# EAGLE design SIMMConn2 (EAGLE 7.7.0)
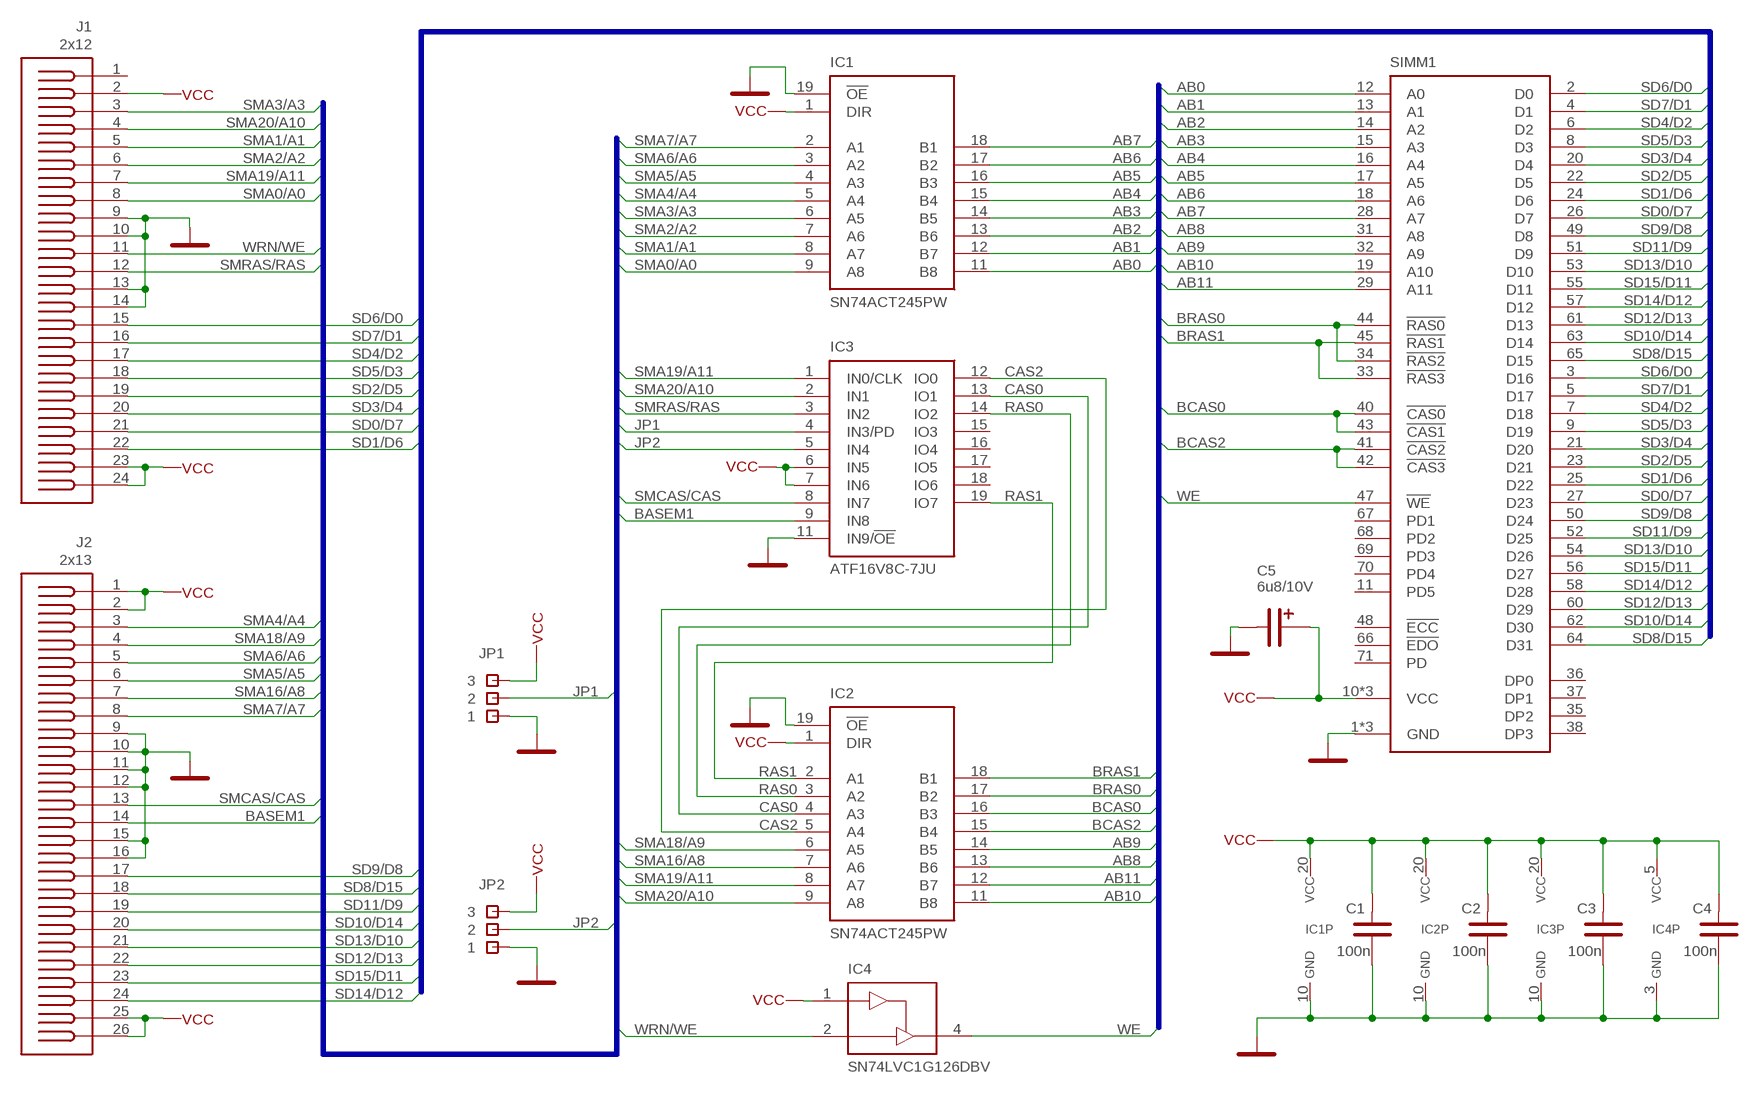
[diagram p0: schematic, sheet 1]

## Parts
C1  100n  CK-SMD-0805  [CK-0805]
C2  100n  CK-SMD-0805  [CK-0805]
C3  100n  CK-SMD-0805  [CK-0805]
C4  100n  CK-SMD-0805  [CK-0805]
C5  6u8/10V  CT-SMD-B  [CT-SMD-B]
IC1  SN74ACT245PW  74245-PW  [TSSOP20]
IC2  SN74ACT245PW  74245-PW  [TSSOP20]
IC3  ATF16V8C-7JU  ATF16V8C  [PLCC20SKT]
IC4  SN74LVC1G126DBV  74-1G126DBV  [SOT23-5]
J1  2x12  20-Z2R24T  [20-Z2R24T]
J2  2x13  20-Z2R26T  [20-Z2R26T]
JP1  JMP1-3  [JMP3-1]
JP2  JMP1-3  [JMP3-1]
SIMM1  SIMM72  [SIMM72A]

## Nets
AB0: IC1.11(B8) SIMM1.12(A0)
AB1: IC1.12(B7) SIMM1.13(A1)
AB2: IC1.13(B6) SIMM1.14(A2)
AB3: IC1.14(B5) SIMM1.15(A3)
AB4: IC1.15(B4) SIMM1.16(A4)
AB5: IC1.16(B3) SIMM1.17(A5)
AB6: IC1.17(B2) SIMM1.18(A6)
AB7: IC1.18(B1) SIMM1.28(A7)
AB8: IC2.13(B6) SIMM1.31(A8)
AB9: IC2.14(B5) SIMM1.32(A9)
AB10: IC2.11(B8) SIMM1.19(A10)
AB11: IC2.12(B7) SIMM1.29(A11)
BASEM1: IC3.9(IN8) J2.14
BCAS0: IC2.16(B3) SIMM1.40(!CAS0) SIMM1.43(!CAS1)
BCAS2: IC2.15(B4) SIMM1.41(!CAS2) SIMM1.42(!CAS3)
BRAS0: IC2.17(B2) SIMM1.34(!RAS2) SIMM1.44(!RAS0)
BRAS1: IC2.18(B1) SIMM1.33(!RAS3) SIMM1.45(!RAS1)
CAS0: IC2.4(A3) IC3.13(IO1)
CAS2: IC2.5(A4) IC3.12(IO0)
GND: C1.1 C2.1 C3.1 C4.1 C5.K IC1.10(GND) IC1.19(!OE) IC2.10(GND) IC2.19(!OE) IC3.10(GND) IC3.11(IN9/!OE) IC4.3(GND) J1.9 J1.10 J1.13 J1.14 J2.9 J2.10 J2.11 J2.12 J2.15 J2.16 JP1.1 JP2.1 SIMM1.1(GND) SIMM1.39(GND) SIMM1.72(GND)
JP1: IC3.4(IN3/PD) JP1.2
JP2: IC3.5(IN4) JP2.2
RAS0: IC2.3(A2) IC3.14(IO2)
RAS1: IC2.2(A1) IC3.19(IO7)
SD0/D7: J1.21 SIMM1.26(D7) SIMM1.27(D23)
SD1/D6: J1.22 SIMM1.24(D6) SIMM1.25(D22)
SD2/D5: J1.19 SIMM1.22(D5) SIMM1.23(D21)
SD3/D4: J1.20 SIMM1.20(D4) SIMM1.21(D20)
SD4/D2: J1.17 SIMM1.6(D2) SIMM1.7(D18)
SD5/D3: J1.18 SIMM1.8(D3) SIMM1.9(D19)
SD6/D0: J1.15 SIMM1.2(D0) SIMM1.3(D16)
SD7/D1: J1.16 SIMM1.4(D1) SIMM1.5(D17)
SD8/D15: J2.18 SIMM1.64(D31) SIMM1.65(D15)
SD9/D8: J2.17 SIMM1.49(D8) SIMM1.50(D24)
SD10/D14: J2.20 SIMM1.62(D30) SIMM1.63(D14)
SD11/D9: J2.19 SIMM1.51(D9) SIMM1.52(D25)
SD12/D13: J2.22 SIMM1.60(D29) SIMM1.61(D13)
SD13/D10: J2.21 SIMM1.53(D10) SIMM1.54(D26)
SD14/D12: J2.24 SIMM1.57(D12) SIMM1.58(D28)
SD15/D11: J2.23 SIMM1.55(D11) SIMM1.56(D27)
SMA0/A0: IC1.9(A8) J1.8
SMA1/A1: IC1.8(A7) J1.5
SMA2/A2: IC1.7(A6) J1.6
SMA3/A3: IC1.6(A5) J1.3
SMA4/A4: IC1.5(A4) J2.3
SMA5/A5: IC1.4(A3) J2.6
SMA6/A6: IC1.3(A2) J2.5
SMA7/A7: IC1.2(A1) J2.8
SMA16/A8: IC2.7(A6) J2.7
SMA18/A9: IC2.6(A5) J2.4
SMA19/A11: IC2.8(A7) IC3.1(IN0/CLK) J1.7
SMA20/A10: IC2.9(A8) IC3.2(IN1) J1.4
SMCAS/CAS: IC3.8(IN7) J2.13
SMRAS/RAS: IC3.3(IN2) J1.12
VCC: C1.2 C2.2 C3.2 C4.2 C5.A IC1.1(DIR) IC1.20(VCC) IC2.1(DIR) IC2.20(VCC) IC3.6(IN5) IC3.7(IN6) IC3.20(VCC) IC4.1(OE) IC4.5(VCC) J1.2 J1.23 J1.24 J2.1 J2.2 J2.25 J2.26 JP1.3 JP2.3 SIMM1.10(VCC) SIMM1.30(VCC) SIMM1.59(VCC)
WE: IC4.4(Y) SIMM1.47(!WE)
WRN/WE: IC4.2(A) J1.11
Unconnected: IC3.15(IO3) IC3.16(IO4) IC3.17(IO5) IC3.18(IO6) J1.1 SIMM1.11(PD5) SIMM1.35(DP2) SIMM1.36(DP0) SIMM1.37(DP1) SIMM1.38(DP3) SIMM1.48(!ECC) SIMM1.66(!EDO) SIMM1.67(PD1) SIMM1.68(PD2) SIMM1.69(PD3) SIMM1.70(PD4) SIMM1.71(PD)

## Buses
D:SD6/D0,SD7/D1,SD4/D2,SD5/D3,SD2/D5,SD3/D4,SD0/D7,SD1/D6,SD9/D8,SD8/D15,SD11/D9,SD10/D14,SD13/D10,SD12/D13,SD15/D11,SD14/D12
A:SMA3/A3,SMA20/A10,SMA1/A1,SMA2/A2,SMA19/A11,SMA0/A0,WRN/WE,SMRAS/RAS,SMA4/A4,SMA18/A9,SMA6/A6,SMA5/A5,SMA16/A8,SMA7/A7,SMCAS/CAS,BASEM1,PD1,PD2,JP1,JP2
B:AB[0..11],BCAS0,BCAS2,BRAS0,BRAS1,WE

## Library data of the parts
C1-C4 = PASIV:CK-SMD: SMD keramické vícevrstvé kondenzátory
C5 = PASIV:CT-SMD: SMD tantalové kondenzátory
IC1 IC2 = IC:74245
IC3 = MEMORY:ATF16V8C
IC4 = IC:74-1G126
J1 = CONNEC:20-Z2R24T
J2 = CONNEC:20-Z2R26T
JP1 JP2 = KONSTR:JMP1-3
SIMM1 = CONNEC:SIMM72

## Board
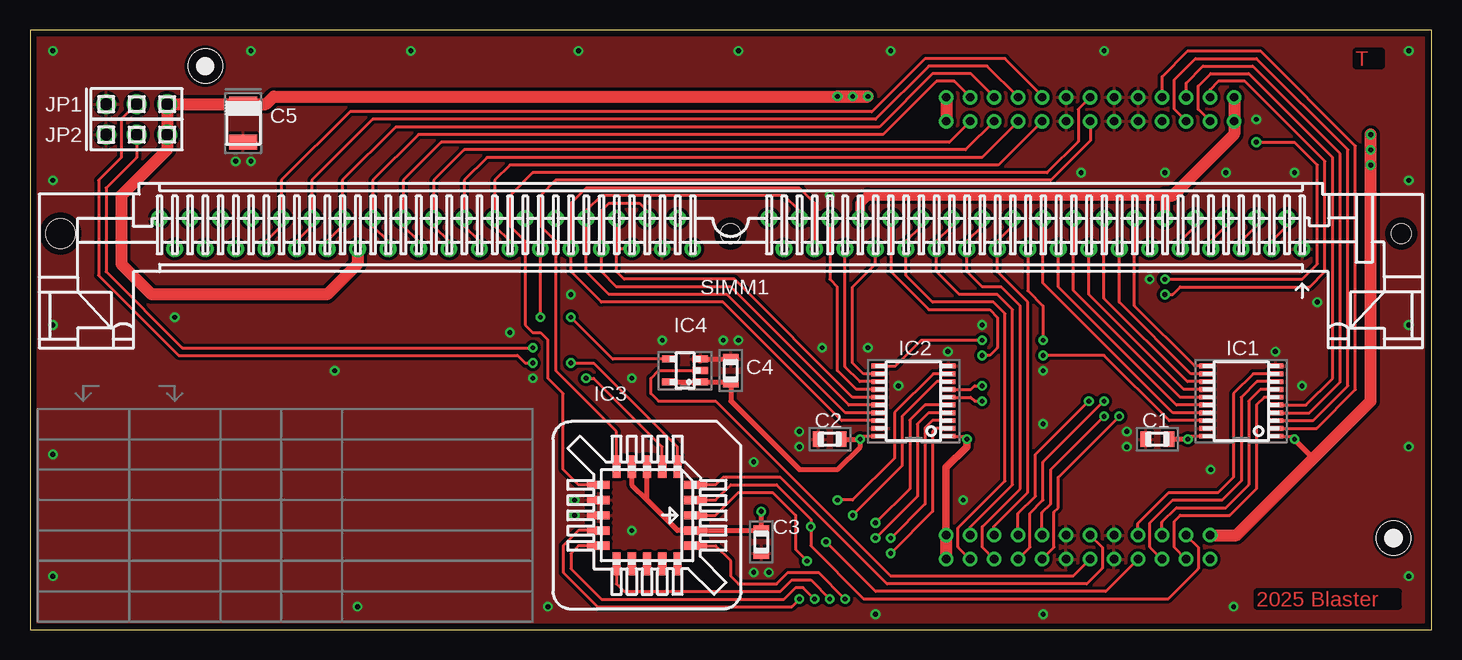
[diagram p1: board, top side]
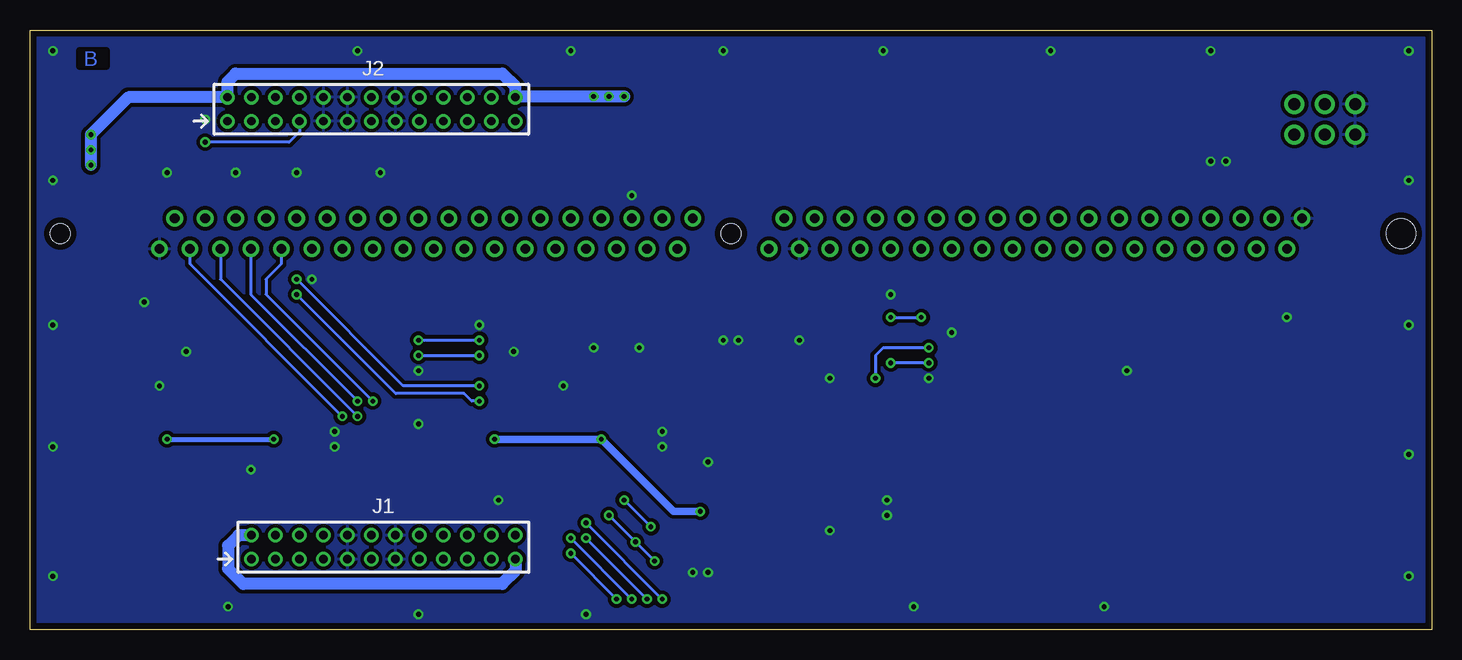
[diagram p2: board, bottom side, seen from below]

Size 116.84 x 50 mm. Coordinates in mm from the lower left corner, seen from the top.
Outline: 0,0 116.84,0 116.84,50 0,50 0,0
Copper layers (1*16): Top 0.035mm / dielectric 1.5mm / Bottom 0.035mm
Design rules "default *": minimum track width 10mil, minimum drill 15mil, track to track 8mil, track to pad 8mil, pad to pad 8mil, via to via 8mil, smd to smd 8mil, copper to edge 20mil, drill to drill 8mil, minimum pad ring 10mil, minimum via ring 8mil, stop-mask expansion 0mil, vias tented up to drill 20mil, thermal gap 10mil
tRestrict: area 110.5,47 to 112.7,48.3
bRestrict: area 110.5,47 to 112.7,48.3

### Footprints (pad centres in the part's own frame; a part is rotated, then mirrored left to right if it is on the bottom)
CK-0805 = smd 0.889 x 1.295: 1 -0.953,0; 2 0.953,0
CT-SMD-B = smd 1.245 x 2.311: A -1.587,0; K 1.587,0
TSSOP20 = smd 0.4 x 1.2: 1 -2.925,-2.9; 2 -2.275,-2.9; 3 -1.625,-2.9; 4 -0.975,-2.9; 5 -0.325,-2.9; 6 0.325,-2.9; 7 0.975,-2.9; 8 1.625,-2.9; 9 2.275,-2.9; 10 2.925,-2.9; 11 2.925,2.9; 12 2.275,2.9; 13 1.625,2.9; 14 0.975,2.9; 15 0.325,2.9; 16 -0.325,2.9; 17 -0.975,2.9; 18 -1.625,2.9; 19 -2.275,2.9; 20 -2.925,2.9
PLCC20SKT = smd 0.7 x 1.91: 1 0,4.06; 2 -1.27,4.06; 3 -2.54,4.06; 9 -2.54,-4.06; 10 -1.27,-4.06; 11 0,-4.06; 12 1.27,-4.06; 13 2.54,-4.06; 19 2.54,4.06; 20 1.27,4.06 | smd 1.91 x 0.7: 4 -4.06,2.54; 5 -4.06,1.27; 6 -4.06,0; 7 -4.06,-1.27; 8 -4.06,-2.54; 14 4.06,-2.54; 15 4.06,-1.27; 16 4.06,0; 17 4.06,1.27; 18 4.06,2.54
SOT23-5 = smd 0.584 x 1.27: 1 0.953,1.27; 2 0,1.27; 3 -0.953,1.27; 4 -0.953,-1.27; 5 0.953,-1.27
20-Z2R24T = drill 0.7 pad 1.2: 1 0,0; 2 0,-2; 3 -2,0; 4 -2,-2; 5 -4,0; 6 -4,-2; 7 -6,0; 8 -6,-2; 9 -8,0; 10 -8,-2; 11 -10,0; 12 -10,-2; 13 -12,0; 14 -12,-2; 15 -14,0; 16 -14,-2; 17 -16,0; 18 -16,-2; 19 -18,0; 20 -18,-2; 21 -20,0; 22 -20,-2; 23 -22,0; 24 -22,-2
20-Z2R26T = drill 0.7 pad 1.2: 1 0,0; 2 0,-2; 3 -2,0; 4 -2,-2; 5 -4,0; 6 -4,-2; 7 -6,0; 8 -6,-2; 9 -8,0; 10 -8,-2; 11 -10,0; 12 -10,-2; 13 -12,0; 14 -12,-2; 15 -14,0; 16 -14,-2; 17 -16,0; 18 -16,-2; 19 -18,0; 20 -18,-2; 21 -20,0; 22 -20,-2; 23 -22,0; 24 -22,-2; 25 -24,0; 26 -24,-2
JMP3-1 = drill 1 pad 1.676: 1 0,0; 2 2.54,0; 3 5.08,0
SIMM72A = drill 0.8 pad 1.4: 1 0,0; 2 -1.27,2.54; 3 -2.54,0; 4 -3.81,2.54; 5 -5.08,0; 6 -6.35,2.54; 7 -7.62,0; 8 -8.89,2.54; 9 -10.16,0; 10 -11.43,2.54; 11 -12.7,0; 12 -13.97,2.54; 13 -15.24,0; 14 -16.51,2.54; 15 -17.78,0; 16 -19.05,2.54; 17 -20.32,0; 18 -21.59,2.54; 19 -22.86,0; 20 -24.13,2.54; 21 -25.4,0; 22 -26.67,2.54; 23 -27.94,0; 24 -29.21,2.54; 25 -30.48,0; 26 -31.75,2.54; 27 -33.02,0; 28 -34.29,2.54; 29 -35.56,0; 30 -36.83,2.54; 31 -38.1,0; 32 -39.37,2.54; 33 -40.64,0; 34 -41.91,2.54; 35 -43.18,0; 36 -44.45,2.54; 37 -50.8,0; 38 -52.07,2.54; 39 -53.34,0; 40 -54.61,2.54; 41 -55.88,0; 42 -57.15,2.54; 43 -58.42,0; 44 -59.69,2.54; 45 -60.96,0; 46 -62.23,2.54; 47 -63.5,0; 48 -64.77,2.54; 49 -66.04,0; 50 -67.31,2.54; 51 -68.58,0; 52 -69.85,2.54; 53 -71.12,0; 54 -72.39,2.54; 55 -73.66,0; 56 -74.93,2.54; 57 -76.2,0; 58 -77.47,2.54; 59 -78.74,0; 60 -80.01,2.54; 61 -81.28,0; 62 -82.55,2.54; 63 -83.82,0; 64 -85.09,2.54; 65 -86.36,0; 66 -87.63,2.54; 67 -88.9,0; 68 -90.17,2.54; 69 -91.44,0; 70 -92.71,2.54; 71 -93.98,0; 72 -95.25,2.54 | hole 2.45: -103.51,1.27 | hole 1.65: -47.63,1.27; 8.26,1.27

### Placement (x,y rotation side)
C1  93.98,15.88 0 top
C2  66.67,15.88 0 top
C3  60.96,7.3 90 top
C4  58.42,21.59 270 top
C5  17.78,42.23 270 top
IC1  100.97,19.05 90 top
IC2  73.66,19.05 90 top
IC3  51.44,9.53 270 top
IC4  54.61,21.59 270 top
J1  98.37,5.87 180 bottom
J2  100.38,42.39 180 bottom
JP1  6.35,43.81 0 top
JP2  6.35,41.27 0 top
REF1  [REF-K]  14.61,46.99 0 top
REF2  [REF-K]  113.67,7.62 0 top
SIMM1  106.05,31.75 0 top

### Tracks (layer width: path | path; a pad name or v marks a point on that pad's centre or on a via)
AB0
  Top 0.254: SIMM1.12 92.08,26.99 97.09,21.98 IC1.11
AB1
  Top 0.254: SIMM1.13 90.81,27.3 96.78,21.32 IC1.12
AB2
  Top 0.254: SIMM1.14 89.53,27.62 96.48,20.68 IC1.13
AB3
  Top 0.254: SIMM1.15 88.27,27.94 96.18,20.02 IC1.14
AB4
  Top 0.254: SIMM1.16 87,28.26 95.88,19.38 IC1.15
AB5
  Top 0.254: SIMM1.17 85.72,28.57 95.58,18.73 IC1.16
AB6
  Top 0.254: SIMM1.18 84.45,28.89 95.27,18.07 IC1.17
AB7  (via drill 0.4)
  Top 0.254: v84.45,22.86 89.53,22.86 94.97,17.43 IC1.18 | SIMM1.28 71.75,29.84 74.93,26.67 80.01,26.67 80.64,26.04 80.64,23.5 80.01,22.86 v79.38,22.86
  Bottom 0.254: v84.45,22.86 v79.38,22.86
AB8
  Top 0.254: SIMM1.31 67.94,21.91 69.18,20.68 IC2.13
AB9
  Top 0.254: SIMM1.32 66.67,29.21 67.31,28.57 67.31,21.59 68.88,20.02 IC2.14
AB10  (via drill 0.4)
  Top 0.254: SIMM1.19 83.19,28.26 84.45,26.99 v84.45,24.13 | IC2.11 72.14,21.98 74.3,24.13 v79.38,24.13
  Bottom 0.254: v84.45,24.13 v79.38,24.13
AB11
  Top 0.254: SIMM1.29 70.48,30.48 68.58,28.57 68.58,22.23 69.48,21.32 IC2.12
BASEM1
  Top 0.254: IC3.9 45.72,12.06 44.45,13.34 44.45,19.68 43.18,20.95 43.18,24.13 42.55,24.77 41.91,24.77 41.27,25.4 41.27,32.38 40.01,33.66 40.01,36.2 41.91,38.1 84.77,38.1 87.38,40.7 87.38,43.39 J2.14
BCAS0
  Top 0.254: SIMM1.40 51.44,34.92 50.8,35.56 48.26,35.56 47.62,34.92 SIMM1.43 47.62,29.84 48.9,28.57 58.42,28.57 68.27,18.73 IC2.16
BCAS2
  Top 0.254: 48.9,31.75 48.9,29.84 49.53,29.21 58.74,29.21 68.57,19.38 IC2.15 | 48.9,31.75 SIMM1.42 | SIMM1.41 48.9,31.75
BRAS0
  Top 0.254: SIMM1.34 64.14,34.92 62.87,36.2 47.62,36.2 46.35,34.92 SIMM1.44 46.35,29.84 48.26,27.94 58.1,27.94 67.97,18.07 IC2.17
BRAS1
  Top 0.254: SIMM1.33 65.41,35.56 64.14,36.83 46.35,36.83 45.09,35.56 SIMM1.45 45.09,29.84 47.62,27.3 57.78,27.3 67.67,17.43 IC2.18
CAS0  (via drill 0.4)
  Top 0.254: IC3.13 45.72,6.99 45.09,6.35 45.09,5.08 47.62,2.54 62.87,2.54 63.82,3.49 64.45,3.49 v65.41,2.54 | IC2.4 74.91,18.07 73.98,17.14 73.98,11.11 v70.48,7.62
  Bottom 0.254: v70.48,7.62 v65.41,2.54
CAS2  (via drill 0.4)
  Top 0.254: IC3.12 45.72,8.26 44.45,6.99 44.45,4.76 47.31,1.91 63.5,1.91 v64.14,2.54 | IC2.5 74.61,18.73 73.34,17.46 73.34,11.75 v70.48,8.89
  Bottom 0.254: v70.48,8.89 v64.14,2.54
GND  (via drill 0.4)
  Top 0.406: IC4.3 C4.1
  other vias: 76.52,23.18 91.44,15.24 64.14,16.51 60.33,4.76 45.4,10.79 45.4,9.53 59.05,24.13 45.09,27.94 66.04,23.5 84.45,17.14 106.05,20.32 102.23,42.55 105.41,38.1 99.69,38.1 94.61,38.1 87.63,38.1 114.94,4.45 114.94,25.4 114.94,48.26 1.91,4.45 1.91,25.4 1.91,48.26 27.3,1.91 31.75,48.26 71.75,48.26 41.91,20.95 25.4,21.59 12.06,26.04 18.41,39.05 18.41,48.26 59.05,48.26 89.53,48.26 70.48,1.27 100.33,1.91 50.16,8.26 72.39,20.32 103.82,23.18 52.7,24.13 64.14,15.24 91.44,16.51 40.01,24.77 1.91,14.61 1.91,37.47 45.72,48.26 114.94,37.47 114.94,15.24 84.45,1.27 43.18,1.91 107.31,27.3 17.14,39.05 77.79,10.79 66.67,36.2 61.59,4.76 60.33,13.97 50.16,20.95 57.78,24.13 79.38,25.4 69.85,23.5 84.45,21.59 93.34,29.21 98.42,13.34
  pour Bottom (isolate 0.305): 0.64,0.64 116.2,0.64 116.2,49.36 0.64,49.36
  pour Top (isolate 0.254): 0.64,0.64 116.2,0.64 116.2,49.36 0.64,49.36
JP1  (via drill 0.4)
  Top 0.254: v41.91,22.23 41.27,22.23 40.64,22.86 12.38,22.86 5.71,29.53 5.71,37.47 7.62,39.37 7.62,42.55 JP1.2 | IC3.4 53.98,15.24 46.99,22.23 v45.09,22.23
  Bottom 0.254: v41.91,22.23 v45.09,22.23
JP2  (via drill 0.4)
  Top 0.254: v41.91,23.5 12.7,23.5 6.35,29.84 6.35,36.83 8.89,39.37 JP2.2 | IC3.5 52.7,15.24 46.99,20.95 v46.35,20.95
  Bottom 0.254: v41.91,23.5 45.72,23.5 46.35,22.86 v46.35,20.95
RAS0  (via drill 0.4)
  Top 0.254: IC3.14 48.9,3.81 49.53,3.17 62.55,3.17 63.5,4.13 65.09,4.13 v66.67,2.54 | IC2.3 75.21,17.43 74.61,16.83 74.61,10.48 v71.75,7.62
  Bottom 0.254: v71.75,7.62 v66.67,2.54
RAS1  (via drill 0.4)
  Top 0.254: IC3.19 57.15,6.99 58.42,5.71 58.42,4.45 59.05,3.81 62.23,3.81 63.18,4.76 65.72,4.76 v67.94,2.54 | IC2.2 75.51,16.77 75.25,16.51 75.25,9.84 v71.75,6.35
  Bottom 0.254: v71.75,6.35 v67.94,2.54
SD0/D7
  Top 0.254: SIMM1.26 74.3,33.66 73.03,32.38 SIMM1.27 73.03,29.53 75.25,27.3 80.33,27.3 81.28,26.35 81.28,12.38 77.37,8.47 77.37,6.87 J1.21
SD1/D6
  Top 0.254: J1.22 78.37,8.52 81.92,12.06 81.92,26.67 80.64,27.94 77.47,27.94 75.56,29.84 SIMM1.25 75.56,32.38 76.83,33.66 SIMM1.24
SD2/D5
  Top 0.254: SIMM1.22 79.38,33.66 78.11,32.38 SIMM1.23 78.11,29.84 79.38,28.57 80.96,28.57 82.55,26.99 82.55,11.75 79.38,8.57 79.38,6.87 J1.19
SD3/D4
  Top 0.254: J1.20 80.37,8.62 83.19,11.43 83.19,27.3 80.64,29.84 SIMM1.21 80.64,32.38 81.92,33.66 SIMM1.20
SD4/D2  (via drill 0.4)
  Top 0.254: v89.53,19.05 84.45,13.97 84.45,10.79 83.36,9.7 83.36,6.86 J1.17 | SIMM1.7 98.42,32.38 99.69,33.66 SIMM1.6
  Bottom 0.254: SIMM1.7 98.42,27.94 v89.53,19.05
SD5/D3  (via drill 0.4)
  Top 0.254: J1.18 82.37,9.67 83.82,11.11 83.82,14.61 v88.27,19.05 | SIMM1.9 95.89,32.38 97.16,33.66 SIMM1.8
  Bottom 0.254: SIMM1.9 95.89,30.48 97.16,29.21 97.16,27.94 v88.27,19.05
SD6/D0  (via drill 0.4)
  Top 0.254: v90.81,17.78 85.72,12.7 85.72,10.16 85.37,9.8 85.37,6.86 J1.15 | SIMM1.3 103.5,32.38 104.78,33.66 SIMM1.2
  Bottom 0.254: v90.81,17.78 103.5,30.48 SIMM1.3
SD7/D1  (via drill 0.4)
  Top 0.254: J1.16 84.37,9.76 85.09,10.48 85.09,13.34 v89.53,17.78 | SIMM1.5 100.97,32.38 102.23,33.66 SIMM1.4
  Bottom 0.254: SIMM1.5 100.97,29.21 v89.53,17.78
SD8/D15
  Top 0.254: SIMM1.65 19.68,32.38 20.95,33.66 SIMM1.64 20.95,37.47 26.67,43.18 70.17,43.18 74.61,47.62 81.28,47.62 84.45,44.45 84.4,44.39 J2.18
SD9/D8
  Top 0.254: J2.17 80.72,38.73 40.01,38.73 38.73,37.47 SIMM1.50 38.73,33.66 40.01,32.38 SIMM1.49
SD10/D14
  Top 0.254: J2.20 79.78,46.99 74.93,46.99 70.48,42.55 28.57,42.55 23.5,37.47 SIMM1.62 23.5,33.66 22.23,32.38 SIMM1.63
SD11/D9
  Top 0.254: SIMM1.51 37.47,32.38 36.2,33.66 SIMM1.52 36.2,37.47 38.1,39.37 79.36,39.37 J2.19
SD12/D13
  Top 0.254: SIMM1.61 24.77,32.38 26.04,33.66 SIMM1.60 26.04,37.47 30.48,41.91 70.8,41.91 75.25,46.35 78.42,46.35 J2.22
SD13/D10
  Top 0.254: J2.21 77.99,40.01 36.2,40.01 33.66,37.47 SIMM1.54 33.66,33.66 34.92,32.38 SIMM1.53
SD14/D12
  Top 0.254: J2.24 77.05,45.72 75.56,45.72 71.12,41.27 32.38,41.27 28.57,37.47 SIMM1.58 28.57,33.66 29.84,32.38 SIMM1.57
SD15/D11
  Top 0.254: SIMM1.55 32.38,32.38 31.11,33.66 SIMM1.56 31.11,37.47 34.29,40.64 76.63,40.64 J2.23
SMA0/A0
  Top 0.254: J1.8 92.37,8.87 94.93,11.43 99.06,11.43 100.33,12.7 100.33,19.68 101.97,21.32 IC1.9
SMA1/A1
  Top 0.254: J1.5 93.37,6.87 93.37,8.91 95.25,10.79 99.38,10.79 100.97,12.38 100.97,19.37 102.27,20.68 IC1.8
SMA2/A2
  Top 0.254: J1.6 94.37,8.97 95.57,10.16 99.69,10.16 101.6,12.06 101.6,19.05 102.58,20.02 IC1.7
SMA3/A3
  Top 0.254: J1.3 95.38,6.87 95.38,9.02 95.89,9.53 100.01,9.53 102.23,11.75 102.23,18.73 102.88,19.38 IC1.6
SMA4/A4
  Top 0.254: J2.3 97.38,43.39 97.38,45.31 98.42,46.35 101.6,46.35 108.58,39.37 108.58,20.95 106.36,18.73 IC1.5
SMA5/A5
  Top 0.254: J2.6 96.38,45.58 97.79,46.99 101.92,46.99 109.22,39.69 109.22,20.64 106.66,18.07 IC1.4
SMA6/A6
  Top 0.254: J2.5 95.38,43.4 95.38,45.85 97.16,47.62 102.23,47.62 109.86,40.01 109.86,20.32 106.96,17.43 IC1.3
SMA7/A7
  Top 0.254: J2.8 94.38,46.12 96.52,48.26 102.55,48.26 110.49,40.32 110.49,20 107.26,16.77 IC1.2
SMA16/A8  (via drill 0.4)
  Top 0.254: v94.61,29.21 106.05,29.21 107.31,30.48 107.31,38.73 105.41,40.64 v102.23,40.64 | IC2.7 78.44,20.02 78.74,20.32 v79.38,20.32
  Bottom 0.254: v79.38,20.32 85.72,20.32 v94.61,29.21 | J2.7 94.38,41.51 95.25,40.64 v102.23,40.64
SMA18/A9  (via drill 0.4)
  Top 0.254: v94.61,27.94 95.25,27.94 95.89,28.57 106.68,28.57 107.95,29.84 107.95,39.05 101.28,45.72 99.06,45.72 98.38,45.04 J2.4 | IC2.6 78.42,19.38 78.74,19.05 v79.38,19.05
  Bottom 0.254: v79.38,19.05 80.01,19.05 80.64,19.68 86.36,19.68 v94.61,27.94
SMA19/A11  (via drill 0.4)
  Top 0.254: J1.7 89.68,3.17 70.48,3.17 v66.36,7.3 | IC3.1 57.15,9.53 59.05,11.43 61.91,11.43 63.82,9.53 63.82,6.67 v64.77,5.71 | IC2.8 75.6,20.68 72.71,17.78 72.71,13.65 v68.58,9.53
  Bottom 0.254: v68.58,9.53 v66.36,7.3 v64.77,5.71
SMA20/A10  (via drill 0.4)
  Top 0.254: IC3.2 57.15,10.79 58.42,12.06 62.23,12.06 65.09,9.21 v65.09,8.57 65.09,6.99 69.53,2.54 94.84,2.54 97.38,5.08 97.38,6.86 J1.4 | IC2.9 75.3,21.32 72.07,18.1 72.07,14.29 68.58,10.79 v67.31,10.79
  Bottom 0.254: v67.31,10.79 v65.09,8.57
SMCAS/CAS
  Top 0.254: J2.13 88.38,40.76 85.09,37.47 43.81,37.47 42.55,36.2 42.55,33.66 43.81,32.38 43.81,21.59 48.9,16.51 IC3.8
SMRAS/RAS
  Top 0.254: IC3.3 57.15,12.06 57.78,12.7 62.55,12.7 71.44,3.81 88.09,3.81 89.38,5.11 89.38,6.86 J1.12
VCC  (via drill 0.4)
  Top 0.254: IC1.1 105.16,16.12 v105.41,15.88 | IC1.20 96.77,16.12 v96.52,15.88 | IC2.1 77.86,16.12 v78.11,15.88 | IC2.20 69.47,16.12 v69.22,15.88
  Top 0.406: 51.44,10.79 53.98,8.26 IC3.20 C3.2 v60.96,9.84 | 51.44,10.79 IC3.6 | IC4.5 IC4.1 C4.2 58.42,19.05 64.14,13.34 67.31,13.34 69.22,15.24 v69.22,15.88 C2.2 | IC3.7 50.16,12.06 51.44,10.79 | v105.41,15.88 107,14.29 | v96.52,15.88 C1.2
  Top 0.61: J1.24 76.37,13.51 78.11,15.24 v78.11,15.88
  Top 0.813: SIMM1.30 69.22,35.56 69.85,36.2 94.61,36.2 SIMM1.10
  Top 1.016: J2.26 J2.25 | J2.2 J2.1 100.38,41.33 95.25,36.2 94.61,36.2 | J1.24 J1.23 | v67.31,44.45 20.32,44.45 19.68,43.81 C5.A JP1.3 JP2.3 11.43,40.01 7.62,36.2 7.62,30.48 10.16,27.94 24.77,27.94 27.3,30.48 SIMM1.59 | v67.31,44.45 v68.58,44.45 v69.85,44.45 v67.31,44.45 | v111.76,41.27 v111.76,40.01 v111.76,38.73 111.76,19.05 107,14.29 100.58,7.87 J1.2
  Bottom 0.406: v105.41,15.88 v96.52,15.88
  Bottom 0.61: v78.11,15.88 v69.22,15.88 63.18,9.84 v60.96,9.84
  Bottom 1.016: J1.23 76.37,4.91 77.47,3.81 99.06,3.81 100.33,5.08 100.33,6.99 99.45,7.87 J1.2 | v67.31,44.45 76.32,44.45 J2.26 76.38,45.27 77.47,46.35 99.69,46.35 100.38,45.67 J2.2 108.64,44.39 v111.76,41.27 v111.76,40.01 v111.76,38.73
WE  (via drill 0.4)
  Top 0.254: IC4.4 48.58,22.54 v45.09,26.04 | v42.55,26.04 SIMM1.47
  Bottom 0.254: v45.09,26.04 v42.55,26.04
WRN/WE
  Top 0.254: J1.11 86.95,4.45 71.75,4.45 57.15,19.05 52.39,19.05 51.75,19.68 51.75,20.95 52.39,21.59 IC4.2

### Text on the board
Top: T | 2025 Blaster
Bottom: B
tValues: 1 - 2 - 3
tPotisk: 1-2-3 | SIMMConn2 for | AWE64 Value/Gold | IC3 | Value | Gold | JP1 | JP2 | Note | 4MB | 1-2 | 1-2 | 8MB | 1-2 | 1-2 | Single Sided | 8MB | 8MB | 2-3 | 1-2 | Double Sided | 16MB | 16MB | 1-2 | 2-3 | 2k Refresh | 16MB | 1-2 | 1-2 | 4k Refresh | 32MB | 32MB | 2-3 | 2-3
bPotisk: JLCJLCJLCJLC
